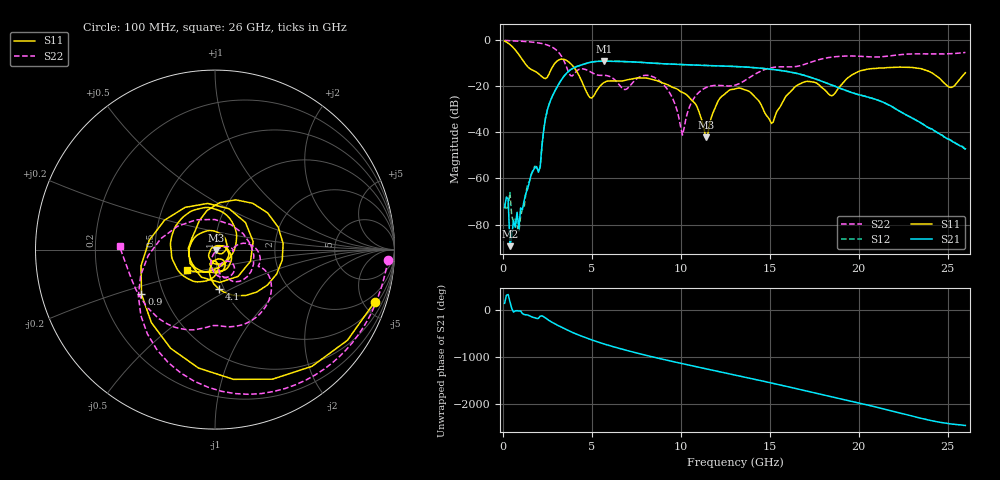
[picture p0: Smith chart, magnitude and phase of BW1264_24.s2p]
!Keysight Technologies,N5245B,MY57181159,A.13.60.06
!Date: Friday, December 18, 2020 23:53:10
!Correction: S11(Full 2 Port(1,2))
!S21(Full 2 Port(1,2))
!S12(Full 2 Port(1,2))
!S22(Full 2 Port(1,2))
!S2P File: Measurements: S11, S21, S12, S22:
# Hz S  dB  R 50
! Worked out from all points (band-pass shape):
!   260 points, 100 MHz to 26 GHz, reference 50 ohm
!   highest |S21| = -9.27 dB at 5.7 GHz (marker M1); lowest = -89.4 dB at 400 MHz (marker M2)
!   |S21| within 3 dB of the highest: 3.957 GHz to 14.45 GHz (10.49 GHz wide, 114 % of centre)
!   lowest |S11| = -42.2 dB at 11.4 GHz (marker M3), VSWR 1.02, Z = 50.6 - j0.455 ohm
!   |S11| at or under -10 dB: 1.224 GHz to 2.95 GHz (1.727 GHz wide, 82.7 % of centre); 3.763 GHz to end of sweep
!   |S22| runs from -41.3 to -0.3 dB; largest |S21 - S12| = 0.00057
!   S11 on the Smith chart (normalised r, x): 100 MHz: 1.27, -6.04; 900 MHz: 0.38, -0.24; 4.1 GHz: 0.95, -0.44; 26 GHz: 0.71, -0.17
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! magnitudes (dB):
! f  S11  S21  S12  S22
! 100 MHz  -0.6  -72.7  -70.9  -0.3
! 300 MHz  -1.5  -68.9  -72.3  -0.4
! 400 MHz  -2.1  -89.4  -66.1  -0.4
! 500 MHz  -2.7  -85.4  -76.2  -0.5
! 900 MHz  -6.4  -81.7  -83.2  -0.6
! 1.7 GHz  -13.3  -56.8  -56.1  -1.1
! 2.1 GHz  -15.3  -54.9  -55.3  -1.5
! 2.6 GHz  -14.8  -28.0  -27.9  -2.6
! 4.1 GHz  -13.0  -11.8  -11.7  -14.0
! 4.5 GHz  -19.1  -10.7  -10.7  -12.6
! 5.7 GHz  -18.5  -9.3  -9.3  -15.4
! 8.8 GHz  -18.1  -10.3  -10.3  -17.7
! 10.1 GHz  -22.8  -10.7  -10.7  -41.3
! 11.4 GHz  -42.2  -11.1  -11.1  -20.8
! 12.1 GHz  -26.5  -11.3  -11.3  -19.8
! 13.1 GHz  -21.2  -11.6  -11.6  -19.6
! 15.1 GHz  -36.2  -12.8  -12.8  -12.1
! 17.4 GHz  -18.2  -16.5  -16.5  -9.5
! 18.5 GHz  -24.2  -19.6  -19.6  -7.5
! 21.7 GHz  -12.0  -28.2  -28.3  -7.0
! 25.2 GHz  -20.6  -43.6  -43.8  -6.0
! 26 GHz  -14.3  -47.2  -47.6  -5.5
